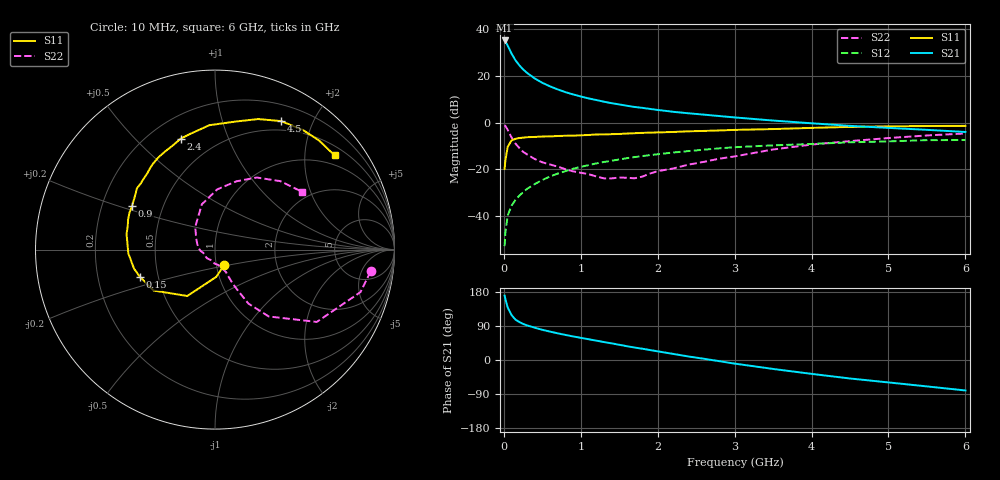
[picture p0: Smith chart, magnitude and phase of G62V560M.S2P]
! SIEMENS Small Signal Semiconductors
! BFG193
! Si NPN RF Bipolar Junction Transistor in SOT223
! VCE = 2.5 V  IC = 60 mA
! Common Emitter S-Parameters:  August  1996
# GHz  S  MA  R  50
!  f  S11  S21  S12  S22
! GHz  MAG  ANG  MAG  ANG  MAG  ANG  MAG  ANG
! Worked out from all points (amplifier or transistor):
!   36 points, 10 MHz to 6 GHz, reference 50 ohm
!   highest |S21| = 35.3 dB at 10 MHz (marker M1)
!   |S21| within 3 dB of that: start of sweep to 61.51 MHz
!   unconditionally stable (mu >= 1): 335.5 MHz to 2.437 GHz
!   at 250 MHz: K = 0.97, MSG = 26.4 dB, |S12| = -30.0 dB
!   at 1.4 GHz: K = 1.06, MAG = 10.9 dB, |S12| = -16.4 dB
!   at 6 GHz: K = 0.92, MSG = 1.7 dB, |S12| = -7.5 dB
!   S11 on the Smith chart (normalised r, x): 10 MHz: 1.09, -0.19; 150 MHz: 0.39, -0.15; 900 MHz: 0.33, +0.22; 2.4 GHz: 0.32, +0.69; 4.5 GHz: 0.39, +1.57; 6 GHz: 0.73, +2.72
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0.01  0.1004 -59.8  57.99 169.8  0.0022 83.4  0.8758 -8.0
0.02  0.1522 -87.5  55.26 161.1  0.0043 78.6  0.8443 -16.3
0.05  0.301 -120.8  44.94 138.6  0.01 67.9  0.6959 -35.4
0.1  0.411 -146.3  30.35 118.6  0.0163 68.8  0.4781 -51.2
0.15  0.4454 -160.1  21.89 106.8  0.0215 66.0  0.3544 -58.2
0.2  0.4638 -166.9  17.07 100.4  0.0266 69.0  0.2854 -60.0
0.25  0.4723 -172.9  13.86 95.3  0.0317 69.0  0.2349 -61.7
0.3  0.4833 -177.4  11.72 91.4  0.0373 70.0  0.2072 -62.6
0.4  0.4894 175.7  8.889 85.4  0.0474 69.8  0.1645 -63.5
0.5  0.5004 170.0  7.127 79.6  0.058 68.9  0.1396 -64.0
0.6  0.5033 165.1  5.981 75.0  0.0693 67.5  0.1254 -66.1
0.7  0.5123 160.9  5.146 70.4  0.0799 66.3  0.1128 -69.8
0.9  0.5217 152.4  4.014 62.2  0.1014 62.4  0.0892 -76.8
1.1  0.539 145.4  3.302 54.8  0.1213 58.7  0.0777 -92.2
1.3  0.5538 138.4  2.805 47.5  0.1419 54.4  0.0631 -109.8
1.6  0.5797 128.7  2.288 36.4  0.1714 47.5  0.0649 -143.5
2.2  0.6259 112.1  1.701 16.2  0.2265 33.4  0.1027 163.5
2.4  0.6472 107.1  1.578 9.3  0.2431 29.2  0.1243 148.1
3.5  0.7228 80.8  1.102 -23.6  0.323 1.6  0.263 106.1
4.5  0.805 62.8  0.847 -48.8  0.3754 -18.6  0.3983 72.7
5.5  0.8402 46.2  0.696 -69.7  0.4174 -41.9  0.5269 46.4
6  0.8482 38.2  0.626 -80.4  0.4208 -55.3  0.5815 33.7
